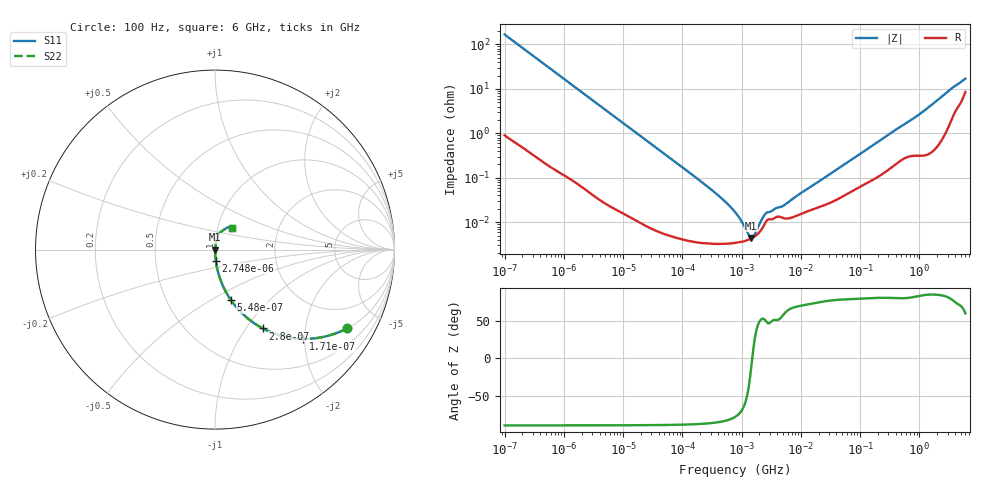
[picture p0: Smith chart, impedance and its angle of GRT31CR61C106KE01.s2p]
!Murata Part Number: GRT31CR61C106KE01
!These Parameters are Measured in Series Mode Connection
!Data Generated on Jun 19, 2026
!  o--ll--o
!Port1  Port2
!  o------o
!Operation Temp=25[degC], DC Bias Voltage=0[V]
!Freq. Start=100[Hz] Stop=6[GHz] 401[Steps]
# Hz S RI R 50
!Freq.(Hz) S11(Real) S11(Imag) S21(Real) S21(Imag) S12(Real) S12(Imag) S22(Real) S22(Imag)
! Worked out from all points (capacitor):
!   401 points, 100 Hz to 6 GHz, reference 50 ohm
!   read as one part in series: C = 9.47 uF near 109 Hz
!   lowest |Z| = 4.4 mohm at 1.45 MHz (marker M1)
!   series resonance near 1.514 MHz, so ESL is about 1.2 nH
!   S11 on the Smith chart (normalised r, x): 100 Hz: 1.02, -3.36; 171 Hz: 1.01, -1.97; 280 Hz: 1.01, -1.20; 548 Hz: 1.00, -0.62; 2.748 kHz: 1.00, -0.12; 6 GHz: 1.17, +0.29
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100  0.7369 -0.4376  0.2631 0.4376  0.2631 0.4376  0.7369 -0.4376
171  0.4913 -0.4971  0.5087 0.4971  0.5087 0.4971  0.4913 -0.4971
280  0.2669 -0.4394  0.7331 0.4394  0.7331 0.4394  0.2669 -0.4394
548  0.0881 -0.2804  0.9119 0.2804  0.9119 0.2804  0.0881 -0.2804
1026  0.0275 -0.1603  0.9725 0.1603  0.9725 0.1603  0.0275 -0.1603
2008  0.00771 -0.0839  0.9923 0.0839  0.9923 0.0839  0.00771 -0.0839
2748  0.00427 -0.0616  0.9957 0.0616  0.9957 0.0616  0.00427 -0.0616
40335  7.83e-05 -0.00427  0.9999 0.00427  0.9999 0.00427  7.83e-05 -0.00427
330837  3.29e-05 -0.0005  1 0.0005  1 0.0005  3.29e-05 -0.0005
541393  3.28e-05 -0.00028  1 0.00028  1 0.00028  3.28e-05 -0.00028
774597  3.41e-05 -0.000167  1 0.000167  1 0.000167  3.41e-05 -0.000167
1059725  3.68e-05 -8.45e-05  1 8.45e-05  1 8.45e-05  3.68e-05 -8.45e-05
1449809  4.28e-05 -1.01e-05  1 1.01e-05  1 1.01e-05  4.28e-05 -1.01e-05
1983483  5.87e-05 6.57e-05  0.9999 -6.57e-05  0.9999 -6.57e-05  5.87e-05 6.57e-05
2713602  0.000112 0.000123  0.9999 -0.000123  0.9999 -0.000123  0.000112 0.000123
5311619  0.000122 0.000211  0.9999 -0.000211  0.9999 -0.000211  0.000122 0.000211
1.555665e7  0.000193 0.00063  0.9998 -0.00063  0.9998 -0.00063  0.000193 0.00063
3.124326e8  0.00166 0.0095  0.9983 -0.0095  0.9983 -0.0095  0.00166 0.0095
9.569533e8  0.00375 0.0252  0.9963 -0.0252  0.9963 -0.0252  0.00375 0.0252
2.562649e9  0.0132 0.0703  0.9868 -0.0703  0.9868 -0.0703  0.0132 0.0703
3.666503e9  0.0328 0.099  0.9672 -0.099  0.9672 -0.099  0.0328 0.099
6e9  0.0953 0.1225  0.9047 -0.1225  0.9047 -0.1225  0.0953 0.1225
